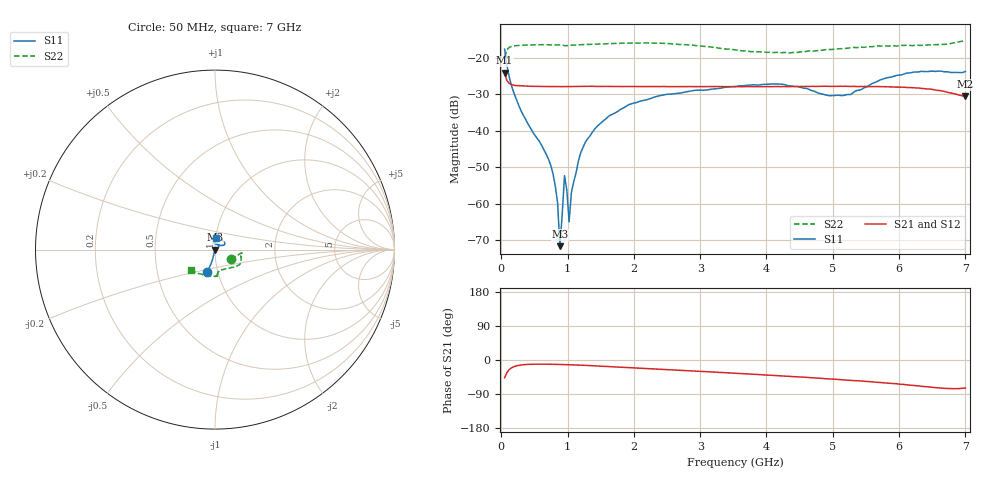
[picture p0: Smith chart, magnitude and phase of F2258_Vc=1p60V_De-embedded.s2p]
! Integrated Device Technology
! Corporate Headquarters
! 6024 Silver Creek Valley Road
! San Jose, CA 95138  USA
! Phone:  1-408-284-8200
! Toll Free:  1-800-223-1366
! Webpage:  http://www.idt.com/
! Timing and RF Division
! 515 Groton Road, Suite 102
! Westford, MA 01886-6024
! Device:  F2258
! Description: Voltage Variable RF Attenuator
! Frequency:  50.0 -  6000.00 MHz
! Package:  3x3 mm Thin QFN Plastic Package: 16 pin
! Ports:  2 RF, 2 DC
!  Pin  1  = NC
!  Pin  2  = NC
!  Pin  3  = RF2  = Port 2
!  Pin  4  = GND
!  Pin  5  = Vdd
!  Pin  6  = NC
!  Pin  7  = VCTRL
!  Pin  8  = NC
!  Pin  9  = GND
!  Pin 10  = RF1  = Port 1
!  Pin 11  = NC
!  Pin 12  = NC
!  Pin 13  = NC
!  Pin 14  = NC
!  Pin 15  = NC
!  Pin 16  = NC
! Vcntrl:  1.600 Volts
! Vdd:  +3.300 Volts
! Current:  1.161 mA
! Data:  The device was measured on a the F2258 evaluation board which has
!  individual transmission lines to the RF pins.  Data was collected
!  using a calibrated network analyzer.  The evaluation board was
!  de-embedded using a TRL calibration technique.
!  The reference plane is the edge of the package pin.
! Misc:  SN 10
!  Action Tracker AT0285
! Date Measured:  2014-12-10
! Date:  2016-01-13  MJV
! Note:
!  Integrated Device Technology supplies this data as a sample of measured
!  data at the package pin for this product.  Your particular data for this
!  product may vary.
!  Data was taken at 25 degrees C.
!  Integrated Device Technology reserves the right to change this data at anytime.
!Freq_(GHz)  S11M_(dB)  S11P_(deg)  S21M_(dB)  S21P_(deg)  S12M_(dB)  S12P_(deg)  S22M_(dB)  S22P_(deg)
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# GHz S dB R 50
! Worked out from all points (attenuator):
!   201 points, 50 MHz to 7 GHz, reference 50 ohm
!   highest |S21| = -24.02 dB at 50 MHz (marker M1); lowest = -30.6 dB at 7 GHz (marker M2)
!   lowest |S11| = -71.7 dB at 884 MHz (marker M3), VSWR 1.00, Z = 50 - j0.0104 ohm
!   |S11| at or under -10 dB: start of sweep to end of sweep
!   |S22| runs from -19.8 to -15.2 dB; largest |S21 - S12| = 0.00045
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0.05  -17.55 -109.4  -24.02 -46.7  -24.01 -46.7  -19.78 -31.3
0.1195  -25.16 -103.9  -26.95 -25.3  -26.96 -25.3  -17.07 -9.9
0.2585  -32.82 -105.1  -27.59 -14.3  -27.67 -14.3  -16.53 -6.8
0.745  -49.45 -104.7  -27.83 -11.2  -27.88 -11.2  -16.38 -11.4
0.8145  -55.21 -99.8  -27.84 -11.5  -27.87 -11.5  -16.39 -12.3
0.84925  -59.83 -93.2  -27.84 -11.6  -27.88 -11.6  -16.41 -12.9
0.884  -71.73 -23.8  -27.85 -11.8  -27.88 -11.8  -16.41 -13.7
0.9535  -52.36 -124.5  -27.84 -12.1  -27.90 -12.1  -16.60 -13.9
0.98825  -56.27 -132.3  -27.84 -12.3  -27.89 -12.3  -16.58 -14.7
1.023  -65.03 -69.5  -27.85 -12.5  -27.85 -12.5  -16.51 -15.3
1.05775  -56.93 -10.3  -27.84 -12.7  -27.87 -12.7  -16.47 -15.6
1.162  -48.42 24.2  -27.80 -13.4  -27.87 -13.3  -16.37 -17.1
1.2315  -44.64 21.5  -27.80 -13.9  -27.85 -13.9  -16.30 -18.0
1.40525  -39.59 21.3  -27.79 -15.5  -27.86 -15.4  -16.20 -20.0
1.61375  -36.09 24.4  -27.80 -17.3  -27.87 -17.3  -16.03 -23.0
2.37825  -30.39 43.1  -27.85 -24.1  -27.91 -24.0  -15.90 -32.1
3.525  -27.83 89.3  -27.86 -34.9  -27.85 -34.9  -17.77 -53.0
4.1505  -27.10 104.0  -27.85 -41.2  -27.84 -41.2  -18.44 -70.7
4.7065  -29.06 94.4  -27.77 -47.0  -27.79 -47.0  -18.07 -80.9
5.2625  -30.06 50.8  -27.81 -53.3  -27.80 -53.3  -17.17 -84.7
5.85325  -25.32 27.5  -27.92 -61.4  -27.91 -61.4  -16.70 -85.9
7  -23.69 83.7  -30.56 -73.8  -30.45 -73.9  -15.16 -139.0
